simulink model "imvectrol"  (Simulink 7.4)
settings: Solver=ode45  StartTime=0.0  StopTime=5  MaxStep=0.001  RelTol=1e-3
undefined symbols (not defined in the file or in its folder): ktune

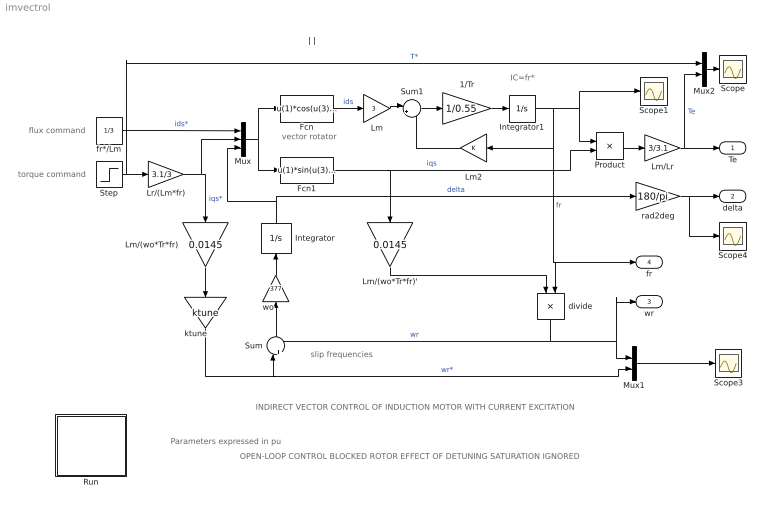
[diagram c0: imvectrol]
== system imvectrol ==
  note: vector rotator
  note: flux command
  note: torque command
  note: INDIRECT VECTOR CONTROL OF INDUCTION MOTOR WITH CURRENT EXCITATION
  note: OPEN-LOOP CONTROL BLOCKED ROTOR EFFECT OF DETUNING SATURATION IGNORED
  note: slip frequencies
  note: | |
  note: Parameters expressed in pu
  note: IC=fr*
  1/Tr : Gain  Gain=1/0.55  ParameterDataType=sfix(16)  ParameterScaling=2^0  OutDataType=sfix(16)  OutScaling=2^0
  Fcn : Fcn  Expr=u(1)*cos(u(3))-u(2)*sin(u(3))
  Fcn1 : Fcn  Expr=u(1)*sin(u(3))+u(2)*cos(u(3))
  Integrator : Integrator
  Integrator1 : Integrator  InitialCondition=1
  Lm : Gain  Gain=3  ParameterDataType=sfix(16)  ParameterScaling=2^0  OutDataType=sfix(16)  OutScaling=2^0
  Lm/(wo*Tr*fr) : Gain  Gain=0.0145  ParameterDataType=sfix(16)  ParameterScaling=2^0  OutDataType=sfix(16)  OutScaling=2^0
  Lm/(wo*Tr*fr)' : Gain  Gain=0.0145  ParameterDataType=sfix(16)  ParameterScaling=2^0  OutDataType=sfix(16)  OutScaling=2^0
  Lm/Lr : Gain  Gain=3/3.1  ParameterDataType=sfix(16)  ParameterScaling=2^0  OutDataType=sfix(16)  OutScaling=2^0
  Lm2 : Gain  ParameterDataType=sfix(16)  ParameterScaling=2^0  OutDataType=sfix(16)  OutScaling=2^0
  Lr/(Lm*fr) : Gain  Gain=3.1/3  ParameterDataType=sfix(16)  ParameterScaling=2^0  OutDataType=sfix(16)  OutScaling=2^0
  Mux : Mux  Inputs=3
  Mux1 : Mux  Inputs=2
  Mux2 : Mux  Inputs=2
  Product : Product  OutDataType=sfix(16)  OutScaling=2^0
  Run : Subsystem
  Scope{,1,3..4} (4 alike) : Scope
  Step : Step  SampleTime=0
  Sum : Sum  Inputs=|+-  OutDataType=sfix(16)  OutScaling=2^0
  Sum1 : Sum  Inputs=|+-  OutDataType=sfix(16)  OutScaling=2^0
  divide : Product  Inputs=*/  OutDataType=sfix(16)  OutScaling=2^0
  fr*/Lm : Constant  Value=1/3  OutDataType=sfix(16)  OutScaling=2^0
  ktune : Gain  Gain=ktune  ParameterDataType=sfix(16)  ParameterScaling=2^0  OutDataType=sfix(16)  OutScaling=2^0
  rad2deg : Gain  Gain=180/pi  ParameterDataType=sfix(16)  ParameterScaling=2^0  OutDataType=sfix(16)  OutScaling=2^0
  wo : Gain  Gain=377  ParameterDataType=sfix(16)  ParameterScaling=2^0  OutDataType=sfix(16)  OutScaling=2^0
  Te : Outport
  delta : Outport  Port=2
  wr : Outport  Port=3
  fr : Outport  Port=4
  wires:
  Mux/1 -> Fcn/1, Fcn1/1
  fr*/Lm/1 -> Mux/1  "ids*"
  Fcn/1 -> Lm/1  "ids"
  wo/1 -> Integrator/1
  Fcn1/1 -> Product/2, Lm/(wo*Tr*fr)'/1  "iqs"
  Sum/1 -> wo/1
  Integrator/1 -> Mux/3, rad2deg/1  "delta"
  Step/1 -> Lr/(Lm*fr)/1, Mux2/1  "T*"
  Lr/(Lm*fr)/1 -> Mux/2, Lm/(wo*Tr*fr)/1  "iqs*"
  Lm/(wo*Tr*fr)/1 -> ktune/1
  ktune/1 -> Mux1/2, Sum/1  "wr*"
  Mux2/1 -> Scope/1
  Product/1 -> Lm/Lr/1
  Lm/(wo*Tr*fr)'/1 -> divide/1
  Mux1/1 -> Scope3/1
  Lm/Lr/1 -> Te/1, Mux2/2  "Te"
  Lm/1 -> Sum1/1
  Sum1/1 -> 1/Tr/1
  1/Tr/1 -> Integrator1/1
  Lm2/1 -> Sum1/2
  Integrator1/1 -> Product/1, Scope1/1, Lm2/1, divide/2, fr/1  "fr"
  divide/1 -> Sum/2, Mux1/1, wr/1  "wr"
  rad2deg/1 -> delta/1, Scope4/1

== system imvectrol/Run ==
  note: Edit to modify the parameters
  note: Double click
  note: This demo illustrates the effect of detuning on the vector control of an induction motor
